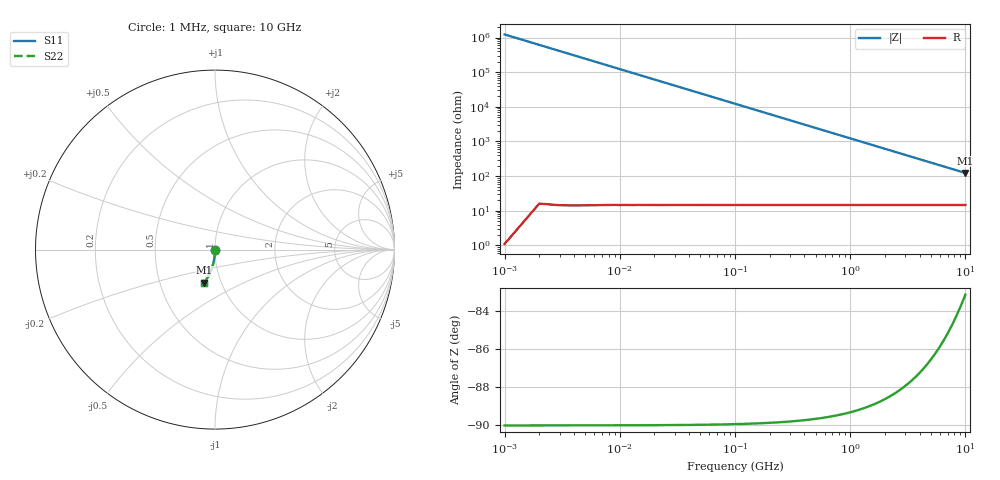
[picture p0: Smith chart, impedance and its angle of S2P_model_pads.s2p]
! Created Wed Nov 08 16:08:49 2017
# hz S ma R 50
! 2 Port Network Data from SP1.SP block
! freq  magS11  angS11  magS21  angS21  magS12  angS12  magS22  angS22
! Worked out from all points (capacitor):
!   10000 points, 1 MHz to 10 GHz, reference 50 ohm
!   read as one part in shunt: C = 130 fF near 51 MHz
!   lowest |Z| = 124 ohm at 10 GHz (marker M1)
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1000000  2.038e-05 -90.0  1 -0.0  1 -0.0  2.038e-05 -90.0
2.5e7  0.0005096 -90.0  1 -0.0  1 -0.0  0.0005096 -90.0
5.7e7  0.001162 -90.1  1 -0.1  1 -0.1  0.001162 -90.1
6.3e7  0.001284 -90.1  1 -0.1  1 -0.1  0.001284 -90.1
8.1e7  0.001651 -90.2  1 -0.1  1 -0.1  0.001651 -90.2
1.04e8  0.00212 -90.2  1 -0.1  1 -0.1  0.00212 -90.2
1.44e8  0.002935 -90.3  1 -0.2  1 -0.2  0.002935 -90.3
1.94e8  0.003954 -90.4  1 -0.2  1 -0.2  0.003954 -90.4
2.56e8  0.005218 -90.5  1 -0.3  1 -0.3  0.005218 -90.5
3.3e8  0.006726 -90.6  1 -0.4  1 -0.4  0.006726 -90.6
4.26e8  0.008683 -90.8  0.9999 -0.5  0.9999 -0.5  0.008683 -90.8
5.4e8  0.01101 -91.0  0.9999 -0.6  0.9999 -0.6  0.01101 -91.0
6.72e8  0.01369 -91.2  0.9998 -0.8  0.9998 -0.8  0.01369 -91.2
8.25e8  0.01681 -91.5  0.9997 -1.0  0.9997 -1.0  0.01681 -91.5
1.197e9  0.02438 -92.2  0.9994 -1.4  0.9994 -1.4  0.02438 -92.2
1.668e9  0.03395 -93.1  0.9987 -1.9  0.9987 -1.9  0.03395 -93.1
2.406e9  0.04889 -94.5  0.9974 -2.8  0.9974 -2.8  0.04889 -94.5
3.334e9  0.06757 -96.2  0.995 -3.9  0.995 -3.9  0.06757 -96.2
5.001e9  0.1006 -99.2  0.9889 -5.8  0.9889 -5.8  0.1006 -99.2
6.667e9  0.1328 -102.2  0.9806 -7.6  0.9806 -7.6  0.1328 -102.2
8.334e9  0.164 -105.1  0.9703 -9.4  0.9703 -9.4  0.164 -105.1
1e10  0.1939 -107.9  0.9582 -11.1  0.9582 -11.1  0.1939 -107.9
